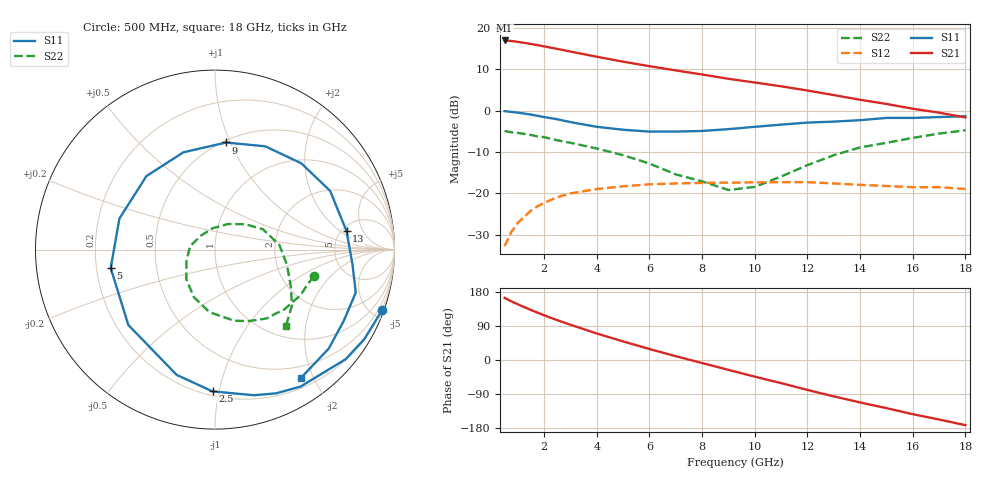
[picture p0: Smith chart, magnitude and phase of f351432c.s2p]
!ATF-35143
!S-PARAMETERS at Vds=2V  Id=15mA.  LAST UPDATED 06-3-99
# ghz s ma r 50
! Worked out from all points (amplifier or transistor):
!   23 points, 500 MHz to 18 GHz, reference 50 ohm
!   highest |S21| = 17.0 dB at 500 MHz (marker M1)
!   |S21| within 3 dB of that: start of sweep to 3.249 GHz
!   unconditionally stable (mu >= 1): 7.831 GHz to end of sweep
!   at 1.5 GHz: K = 0.26, MSG = 20.2 dB, |S12| = -24.2 dB
!   at 7 GHz: K = 0.93, MSG = 13.7 dB, |S12| = -17.6 dB
!   at 18 GHz: K = 1.37, MAG = 5.0 dB, |S12| = -18.9 dB
!   lowest NFmin = 0.10 dB at 500 MHz
!   S11 on the Smith chart (normalised r, x): 500 MHz: 0.17, -5.67; 2.5 GHz: 0.23, -0.96; 5 GHz: 0.26, -0.08; 9 GHz: 0.52, +0.97; 13 GHz: 5.52, +2.51; 18 GHz: 0.33, -1.83
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0.5  0.99 -20.0  7.1 164.0  0.023 78.0  0.57 -15.0
0.75  0.97 -31.0  7 155.0  0.034 71.0  0.55 -21.0
1  0.95 -40.0  6.83 147.0  0.044 65.0  0.54 -28.0
1.5  0.9 -58.0  6.44 132.0  0.062 54.0  0.51 -41.0
1.75  0.87 -67.0  6.23 125.0  0.07 49.0  0.49 -47.0
2  0.84 -75.0  6.02 118.0  0.077 44.0  0.48 -53.0
2.5  0.79 -91.0  5.61 105.0  0.09 35.0  0.44 -65.0
3  0.73 -107.0  5.21 93.0  0.1 27.0  0.41 -75.0
4  0.64 -139.0  4.51 70.0  0.113 11.0  0.35 -95.0
5  0.59 -170.0  3.93 49.0  0.122 -3.0  0.29 -114.0
6  0.56 162.0  3.47 29.0  0.129 -16.0  0.23 -134.0
7  0.56 133.0  3.08 10.0  0.132 -29.0  0.17 -159.0
8  0.57 108.0  2.75 -8.0  0.134 -41.0  0.14 172.0
9  0.6 84.0  2.44 -26.0  0.135 -53.0  0.11 134.0
10  0.64 64.0  2.2 -44.0  0.136 -63.0  0.12 96.0
11  0.68 45.0  1.98 -61.0  0.137 -75.0  0.16 63.0
12  0.72 27.0  1.76 -79.0  0.137 -86.0  0.22 40.0
13  0.74 8.0  1.55 -96.0  0.132 -98.0  0.29 23.0
14  0.77 -6.0  1.36 -112.0  0.127 -108.0  0.36 4.0
15  0.82 -17.0  1.21 -127.0  0.123 -117.0  0.41 -12.0
16  0.82 -29.0  1.06 -143.0  0.119 -127.0  0.47 -26.0
18  0.86 -56.0  0.83 -172.0  0.113 -148.0  0.58 -47.0
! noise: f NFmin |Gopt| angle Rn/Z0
0.5  0.1  0.88  5  0.19
0.9  0.13  0.83  13  0.17
1.5  0.19  0.76  26  0.15
1.8  0.22  0.72  33  0.15
2.5  0.29  0.64  49  0.12
3  0.34  0.58  61  0.07
5  0.56  0.42  117  0.07
6  0.67  0.37  149  0.05
8  0.9  0.33  -144  0.07
10  1.12  0.36  -76  0.23
